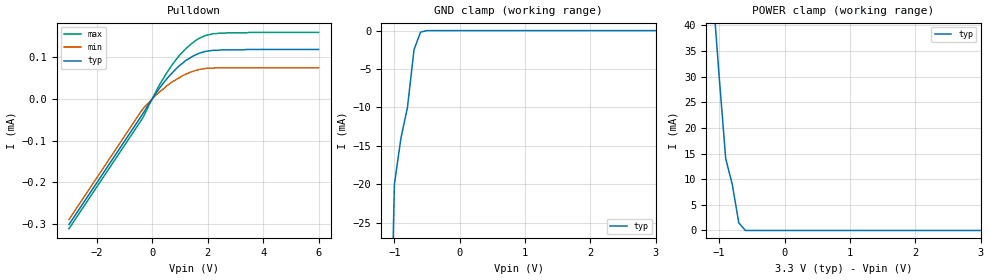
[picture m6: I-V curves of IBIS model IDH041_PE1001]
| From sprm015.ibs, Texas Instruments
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[Model]   IDH041_PE1001
Model_type   Input
Polarity   Non-Inverting
| signals   A, PWRDN, TAP, Y
Vinl = 0.8V
Vinh = 2.0V
|   typ   min   max
C_comp   3.9541p   3.8409p   4.2839p
|   typ   min   max
[Temperature Range]   25.0   0   90
|   typ   min   max
[Voltage Range]   3.3V   3.13V   3.47V
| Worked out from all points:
|   slope of the pulldown table from 0 to 0.495 V, typ, clamps not added: 10.9 kohm
|   GND clamp passes 1 mA (typ) near -0.63 V on its own axis
|   POWER clamp passes 1 mA (typ) near -0.67 V on its own axis
[Pulldown]
|   Voltage   I(typ)   I(min)   I(max)
-3V       -302uA     -290uA     -312uA
-300mV    -32uA      -21uA      -41uA
200mV     20uA       13uA       26uA
500mV     46uA       30uA       60uA
900mV     75uA       48uA       98uA
1.2V      92uA       59uA       120uA
1.4V      100uA      65uA       132uA
1.7V      110uA      71uA       146uA
1.9V      114uA      73uA       152uA
2.2V      117uA      74uA       157uA
3.5V      119uA      75uA       160uA
6V        119uA      75uA       160uA
[GND_clamp]
|   Voltage   I(typ)   I(min)   I(max)
-3V       -900mA     NA         NA
-2V       -400mA     NA         NA
-1V       -20mA      NA         NA
-900mV    -14mA      NA         NA
-800mV    -10mA      NA         NA
-700mV    -2.5mA     NA         NA
-600mV    -200uA     NA         NA
-500mV    0A         NA         NA
3V        0A         NA         NA
[POWER_clamp]
|   Voltage   I(typ)   I(min)   I(max)
-3V       600mA      NA         NA
-2V       200mA      NA         NA
-1V       30mA       NA         NA
-900mV    14mA       NA         NA
-800mV    9mA        NA         NA
-700mV    1.5mA      NA         NA
-600mV    0A         NA         NA
-500mV    0A         NA         NA
3V        0A         NA         NA
